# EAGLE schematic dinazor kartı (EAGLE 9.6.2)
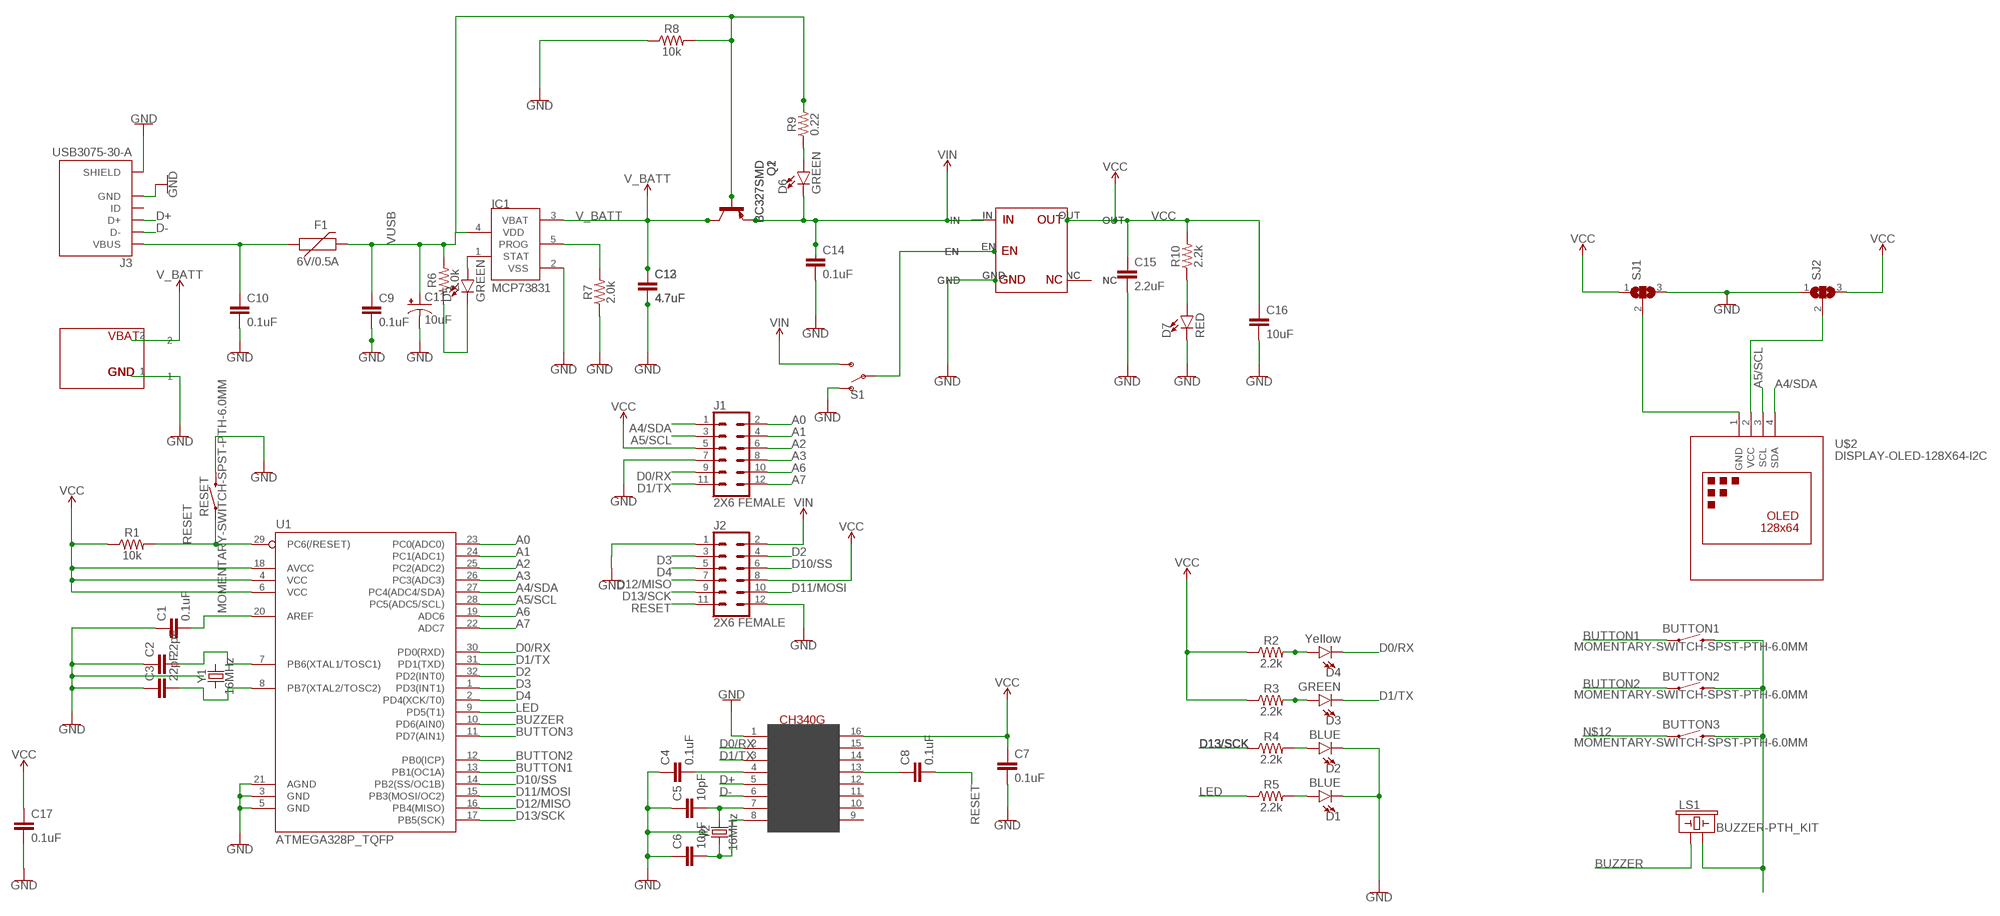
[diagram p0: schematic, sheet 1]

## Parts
BUTTON1  MOMENTARY-SWITCH-SPST-PTH-6.0MM  [TACTILE_SWITCH_PTH_6.0MM]
BUTTON2  MOMENTARY-SWITCH-SPST-PTH-6.0MM  [TACTILE_SWITCH_PTH_6.0MM]
BUTTON3  MOMENTARY-SWITCH-SPST-PTH-6.0MM  [TACTILE_SWITCH_PTH_6.0MM]
C1  0.1uF  0.1UF-0603-25V-(+80/-20%)  [0603]
C2  22pF  22PF-0603-50V-5%  [0603]
C3  22pF  22PF-0603-50V-5%  [0603]
C4  0.1uF  0.1UF-0603-25V-(+80/-20%)  [0603]
C5  10pF  10PF-0603-50V-5%  [0603]
C6  10pF  10PF-0603-50V-5%  [0603]
C7  0.1uF  0.1UF-0402-16V-10%  [0402]
C8  0.1uF  0.1UF-0402-16V-10%  [0402]
C9  0.1uF  0.1UF-0402-16V-10%  [0402]
C10  0.1uF  0.1UF-0402-16V-10%  [0402]
C11  10uF  10UF-POLAR-0603-6.3V-20%(TANT)  [0603-POLAR]
C12  4.7uF  4.7UF-1206-16V-(+80/-20%)  [1206]
C13  4.7uF  4.7UF-1206-16V-(+80/-20%)  [1206]
C14  0.1uF  0.1UF-0603-25V-5%  [0603]
C15  2.2uF  2.2UF-0805-25V-(+80/-20%)  [0805]
C16  10uF  10UF-0805-10V-10%  [0805]
C17  0.1uF  0.1UF-0402-16V-10%  [0402]
D1  BLUE  LED-BLUE0603  [LED-0603]
D2  BLUE  LED-BLUE0603  [LED-0603]
D3  GREEN  LED-GREEN0603  [LED-0603]
D4  Yellow  LED-YELLOW0603  [LED-0603]
D5  GREEN  LED-GREEN0603  [LED-0603]
D6  GREEN  LED-GREEN0603  [LED-0603]
D7  RED  LED-RED0603  [LED-0603]
F1  6V/0.5A  PPTC_HALF-AMP  [1206]
IC1  MCP73831  [SOT23-5L]
J1  2X6 FEMALE  CONN_06X2PTH_FEMALE  [2X6]
J2  2X6 FEMALE  CONN_06X2PTH_FEMALE  [2X6]
J3  USB3075-30-A  [GCT_USB3075-30-A]
LS1  BUZZER-PTH_KIT  [BUZZER-12MM-KIT]
Q1  BC327SMD  [SOT23-BEC]
Q2  BC327SMD  [SOT23-BEC]
R1  10k  10KOHM-HORIZ_KIT-1/4W-5%  [AXIAL-0.3-KIT]
R2  2.2k  2.2KOHM-0603-1/10W-1%  [0603]
R3  2.2k  2.2KOHM-0603-1/10W-1%  [0603]
R4  2.2k  2.2KOHM-0603-1/10W-1%  [0603]
R5  2.2k  2.2KOHM-0603-1/10W-1%  [0603]
R6  2.0k  2.0KOHM-0603-1/10W-5%  [0603]
R7  2.0k  2.0KOHM-0603-1/10W-5%  [0603]
R8  10k  10KOHM-0603-1/10W-1%  [0603]
R9  0.22  0.22OHM-0805-1/4W-1%  [0805]
R10  2.2k  2.2KOHM-0603-1/10W-1%  [0603]
RESET  MOMENTARY-SWITCH-SPST-PTH-6.0MM  [TACTILE_SWITCH_PTH_6.0MM]
S1  SWITCH-SPDT-PTH-11.6X4.0MM  [SWITCH_SPDT_PTH_11.6X4.0MM]
SJ1  SJ2W  [SJ_2]
SJ2  SJ2W  [SJ_2]
U1  ATMEGA328P_TQFP  [TQFP32-08]
U$1  CH340G  [SOIC16]
U$2  DISPLAY-OLED-128X64-I2C  [DISPLAY-OLED-128X64-I2C]
U$3  LİPOBATTERY  [LİPOBATTERY]
U$4  3.3V  [3.3V]
U$5  3.3V  [3.3V]
Y1  16MHz  CRYSTAL-16MHZPTH-HC49US  [HC49US]
Y2  16MHz  CRYSTAL-16MHZPTH-HC49US  [HC49US]

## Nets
A0: J1.2 U1.23(PC0(ADC0))
A1: J1.4 U1.24(PC1(ADC1))
A2: J1.6 U1.25(PC2(ADC2))
A3: J1.8 U1.26(PC3(ADC3))
A4/SDA: J1.1 U1.27(PC4(ADC4/SDA)) U$2.4(SDA)
A5/SCL: J1.3 U1.28(PC5(ADC5/SCL)) U$2.3(SCL)
A6: J1.10 U1.19(ADC6)
A7: J1.12 U1.22(ADC7)
BUTTON1: BUTTON1.1 U1.13(PB1(OC1A))
BUTTON2: BUTTON2.1 U1.12(PB0(ICP))
BUTTON3: U1.11(PD7(AIN1))
BUZZER: LS1.+ U1.10(PD6(AIN0))
D0/RX: D4.C J1.9 U1.30(PD0(RXD)) U$1.2(TX)
D1/TX: D3.C J1.11 U1.31(PD1(TXD)) U$1.3(RX)
D2: J2.4 U1.32(PD2(INT0))
D3: J2.3 U1.1(PD3(INT1))
D4: J2.5 U1.2(PD4(XCK/T0))
D10/SS: J2.6 U1.14(PB2(SS/OC1B))
D11/MOSI: J2.10 U1.15(PB3(MOSI/OC2))
D12/MISO: J2.7 U1.16(PB4(MISO))
D13/SCK: J2.9 R4.1 U1.17(PB5(SCK))
D+: J3.3(D+) U$1.5(D+)
D-: J3.2(D-) U$1.6(D-)
GND: C1.1 C2.1 C3.1 C4.1 C5.1 C6.1 C7.2 C9.2 C10.2 C11.- C12.2 C13.2 C14.2 C15.2 C16.2 C17.2 D1.C D2.C D7.C IC1.2(VSS) J1.7 J2.1 J2.12 J3.5(GND) J3.S1(SHIELD) J3.S2(SHIELD) J3.S3(SHIELD) J3.S4(SHIELD) J3.S5(SHIELD) J3.S6(SHIELD) R7.1 R8.1 RESET.3 S1.1(O) SJ1.3 SJ2.1 U1.3(GND) U1.5(GND) U1.21(AGND) U$1.1(GND) U$3.1 U$4.GND U$5.GND
LED: R5.1 U1.9(PD5(T1))
N$1: D3.A R3.2
N$2: C1.2 U1.20(AREF)
N$3: C4.2 U$1.4(V3)
N$4: C2.2 U1.7(PB6(XTAL1/TOSC1))
N$5: C3.2 U1.8(PB7(XTAL2/TOSC2))
N$6: C6.2 U$1.8(XO) Y2.1
N$7: C5.2 U$1.7(XI) Y2.2
N$8: D4.A R2.2
N$9: C8.1 U$1.13(DTR)
N$10: SJ1.2 U$2.1(GND)
N$11: SJ2.2 U$2.2(VCC)
N$12: BUTTON3.1
N$13: D2.A R4.2
N$14: D1.A R5.2
N$17: BUTTON1.3 BUTTON2.3 BUTTON3.3 LS1.-
N$18: C10.1 F1.1 J3.1(VBUS)
N$19: D5.C R6.1
N$20: D5.A IC1.1(STAT)
N$21: D6.A R9.1
N$22: IC1.5(PROG) R7.2
N$23: U$4.IN U$5.IN
N$24: S1.2(P) U$4.EN U$5.EN
N$26: U$4.NC U$5.NC
N$31: D7.A R10.1
RESET: C8.2 J2.11 R1.P$2 RESET.1 U1.29(PC6(/RESET))
V_BATT: C12.1 C13.1 IC1.3(VBAT) Q1.C Q2.C U$3.2
VCC: C7.1 C15.1 C16.1 C17.1 J1.5 J2.8 R1.P$1 R2.1 R3.1 R10.2 SJ1.1 SJ2.3 U1.4(VCC) U1.6(VCC) U1.18(AVCC) U$1.16(VCC) U$4.OUT U$5.OUT
VIN: C14.1 D6.C J2.2 Q1.E Q2.E S1.3(S)
VUSB: C9.1 C11.+ F1.2 IC1.4(VDD) Q1.B Q2.B R6.2 R8.2 R9.2
Unconnected: J3.4(ID) U$1.9(CTS) U$1.10(DSR) U$1.11(RI) U$1.12(DCD) U$1.14(RTS) U$1.15(RS232) Y1.1 Y1.2

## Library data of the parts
BUTTON1-BUTTON3 RESET = SparkFun-Switches:MOMENTARY-SWITCH-SPST: Momentary Switch (Pushbutton) - SPST; PROD_ID: SWCH-08441; SF_SKU: COM-00097
C1 C4 = SparkFun-Capacitors:0.1UF: 0.1µF ceramic capacitors; PROD_ID: CAP-00810
C2 C3 = SparkFun-Capacitors:22PF: 22pF ceramic capacitors; PROD_ID: CAP-07876
C5 C6 = SparkFun-Capacitors:10PF: 10pF ceramic capacitors; PROD_ID: CAP-11812
C7-C10 C17 = SparkFun-Capacitors:0.1UF: 0.1µF ceramic capacitors; PROD_ID: CAP-12416
C11 = SparkFun-Capacitors:10UF-POLAR: 10.0µF polarized capacitors; PROD_ID: CAP-13210
C12 C13 = SparkFun-Capacitors:4.7UF: 4.7µF ceramic capacitors; PROD_ID: CAP-10300
C14 = SparkFun-Capacitors:0.1UF: 0.1µF ceramic capacitors; PROD_ID: CAP-08604
C15 = SparkFun-Capacitors:2.2UF: 2.2µF ceramic capacitors; PROD_ID: CAP-11624
C16 = SparkFun-Capacitors:10UF: 10.0µF ceramic capacitors; PROD_ID: CAP-11330
D1 D2 = SparkFun-LED:LED-BLUE: Blue SMD LED; PROD_ID: DIO-08575
D3 D5 D6 = SparkFun-LED:LED-GREEN: Green SMD LED; PROD_ID: DIO-00821
D4 = SparkFun-LED:LED-YELLOW: Yellow SMD LED; PROD_ID: DIO-09003
D7 = SparkFun-LED:LED-RED: Red SMD LED; PROD_ID: DIO-00819
F1 = SparkFun-Fuses:PPTC: Resettable Fuse PPTC; PROD_ID: RES-08585
IC1 = microchip-update:MCP73831: Miniature Single-Cell, Fully Integrated Li-Ion, Li-Polymer Charge Management Controllers
J1 J2 = SparkFun-Connectors:CONN_06X2: Multi connection point. Often used as Generic Header-pin footprint for 0.1 inch spaced/style header connections On any of the 0.1 inch spaced packages, you can populate with these: Break Away Headers - Straight (PRT-00116) Break Away Male Headers - Right Angle (PRT-00553) Female Headers (PRT-00115)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; PROD_ID: CONN-12423
J3 = USB3075-30-A:USB3075-30-A: Micro USB Receptacle, Type B, 5 Pin, SMT, Horizontal, Bottom Mount (Standart), without Peg, with Outer Shell Stakes Check prices; AVAILABILITY: In Stock; DESCRIPTION: USB - micro B USB 2.0 Receptacle Connector 5 Position Surface Mount, Right Angle; Through Hole, 2.35mm profile, 5 Pins, Horizontal, Bottom mount; MF: Global Connector Technology; MP: USB3075-30-A; PACKAGE: None; PRICE: None; PURCHASE-URL: https://pricing.snapeda.com/search/part/USB3075-30-A/?ref=eda
LS1 = SparkFun-Electromechanical:BUZZER: Buzzer; PROD_ID: COMP-08253; SF_SKU: COM-07950
Q1 Q2 = transistor-pnp:BC327*: PNP Transistror
R1 = SparkFun-Resistors:10KOHM: 10kΩ resistor; PROD_ID: RES-09435
R2-R5 R10 = SparkFun-Resistors:2.2KOHM: 2.2kΩ resistor; PROD_ID: RES-08272
R6 R7 = SparkFun-Resistors:2.0KOHM: 2kΩ resistor; PROD_ID: RES-08296
R8 = SparkFun-Resistors:10KOHM: 10kΩ resistor; PROD_ID: RES-00824
R9 = SparkFun-Resistors:0.22OHM: 0.22Ω resistor; PROD_ID: RES-09883
S1 = SparkFun-Switches:SWITCH-SPDT: Single Pole, Double Throw (SPDT) Switch Single-pole, double-throw (SPDT) switch. Variant Overview SMD-AYZ0202 Surface Mount DPDT Switch (COM-00597) Used on e.g. LilyPad Arduino USB - ATmega32U4 Board PTH-11.6X4.0MM SPDT Mini Power Switch (COM-00102) Used on e.g. SparkFun Simon Says - Through-Hole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; PROD_ID: SWCH-08261; SF_SKU: COM-00102
SJ1 SJ2 = jumper:SJ2W: SMD solder JUMPER
U1 = SparkFun-IC-Microcontroller:ATMEGA328P_TQFP: Popular 328P in QFP Storefront component: ATmega328 - TQFP (COM-13448) Datasheet SparkFun Products SparkFun RedBoard - Programmed with Arduino (DEV-12757) Arduino Pro Mini 328 - 5V/16MHz (DEV-11113) Arduino Pro Mini 328 - 3.3V/8MHz (DEV-11114) SparkFun OpenLog (DEV-13712) SparkFun MicroView - OLED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; PROD_ID: IC-09069
U$1 = usb-serial:CH340G
U$2 = diy-modules:DISPLAY-OLED-128X64-I2C: 128x64 Dot Matrix OLED Module based on SSD1306 chip Variant with I2C interface More details available here: http://www.instructables.com/id/Monochrome-096-i2c-OLED-display-with-arduino-SSD13/ SSD1306 datasheet: https://cdn-shop.adafruit.com/datasheets/SSD1306.pdf Click here to find device on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
U$3 = untitled:LİPOBATTERY
U$4 U$5 = untitled:3.3V
Y1 Y2 = SparkFun-Clocks:CRYSTAL-16MHZ: 16MHz Crystal; PROD_ID: XTAL-08181; SF_ID: COM-00536

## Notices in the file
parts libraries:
SparkFun-IC-Microcontroller: Licensing: Creative Commons ShareAlike 4.0 International - https://creativecommons.org/licenses/by-sa/4.0
diy-modules: Released under the Creative Commons Attribution 4.0 International License: http://creativecommons.org/licenses/by/4.0
